DATA_BLOCK "PMA_DG1_RECV"
TITLE =
VERSION : 0.1


  STRUCT
   i_noStpULoad : BOOL ;	//Indication: No stop in case of underload
   Spare_00_1 : BOOL ;	//Spare
   Spare_00_2 : BOOL ;	//Spare
   Spare_00_3 : BOOL ;	//Spare
   Spare_00_4 : BOOL ;	//Spare
   Spare_00_5 : BOOL ;	//Spare
   Spare_00_6 : BOOL ;	//Spare
   Spare_00_7 : BOOL ;	//Spare
   i_Gen_run : BOOL ;	//Indication: DG running
   i_Gen_stp : BOOL ;	//Indication: DG not running
   i_Gen_strtAct : BOOL ;	//Indication: DG starting
   i_Gen_stpAct : BOOL ;	//Indication: DG stopping
   Spare_01_4 : BOOL ;	//Spare
   i_Gen_RdyStrt : BOOL ;	//Indication: DG ready for start
   Spare_01_6 : BOOL ;	//Spare
   Spare_01_7 : BOOL ;	//Spare
   i_GenBrkClse : BOOL ;	//Indication: Generator breaker closed
   i_GenBrkOpn : BOOL ;	//Indication: Generator breaker open
   i_GenBrkClseAct : BOOL ;	//Indication: Generator breaker closing active
   Spare_02_3 : BOOL ;	//Spare
   Spare_02_4 : BOOL ;	//Spare
   i_GenBrk_chrg : BOOL ;	//Indication: Generator spring in charge
   i_GenBrk_rdy : BOOL ;	//Indication: Generator breaker ready
   Spare_02_7 : BOOL ;	//Spare
   Spare_03_0 : BOOL ;	//Spare
   Spare_03_1 : BOOL ;	//Spare
   Spare_03_2 : BOOL ;	//Spare
   Spare_03_3 : BOOL ;	//Spare
   Spare_03_4 : BOOL ;	//Spare
   Spare_03_5 : BOOL ;	//Spare
   Spare_03_6 : BOOL ;	//Spare
   i_LifeFlag : BOOL ;	//Indication: PMS unit is alive (5sec pulse, 10 sec period)
   Spare_04_0 : BOOL ;	//Spare
   Spare_04_1 : BOOL ;	//Spare
   Spare_04_2 : BOOL ;	//Spare
   Spare_04_3 : BOOL ;	//Spare
   Spare_04_4 : BOOL ;	//Spare
   Spare_04_5 : BOOL ;	//Spare
   Spare_04_6 : BOOL ;	//Spare
   Spare_04_7 : BOOL ;	//Spare
   Spare_05_0 : BOOL ;	//Spare
   Spare_05_1 : BOOL ;	//Spare
   Spare_05_2 : BOOL ;	//Spare
   Spare_05_3 : BOOL ;	//Spare
   Spare_05_4 : BOOL ;	//Spare
   Spare_05_5 : BOOL ;	//Spare
   Spare_05_6 : BOOL ;	//Spare
   Spare_05_7 : BOOL ;	//Spare
   Spare_06_0 : BOOL ;	//Spare
   Spare_06_1 : BOOL ;	//Spare
   Spare_06_2 : BOOL ;	//Spare
   Spare_06_3 : BOOL ;	//Spare
   Spare_06_4 : BOOL ;	//Spare
   Spare_06_5 : BOOL ;	//Spare
   Spare_06_6 : BOOL ;	//Spare
   Spare_06_7 : BOOL ;	//Spare
   Spare_07_0 : BOOL ;	//Spare
   Spare_07_1 : BOOL ;	//Spare
   Spare_07_2 : BOOL ;	//Spare
   Spare_07_3 : BOOL ;	//Spare
   Spare_07_4 : BOOL ;	//Spare
   Spare_07_5 : BOOL ;	//Spare
   Spare_07_6 : BOOL ;	//Spare
   Spare_07_7 : BOOL ;	//Spare
   Spare_08_0 : BOOL ;	//Spare
   Spare_08_1 : BOOL ;	//Spare
   Spare_08_2 : BOOL ;	//Spare
   Spare_08_3 : BOOL ;	//Spare
   Spare_08_4 : BOOL ;	//Spare
   Spare_08_5 : BOOL ;	//Spare
   Spare_08_6 : BOOL ;	//Spare
   Spare_08_7 : BOOL ;	//Spare
   Spare_09_0 : BOOL ;	//Spare
   Spare_09_1 : BOOL ;	//Spare
   Spare_09_2 : BOOL ;	//Spare
   Spare_09_3 : BOOL ;	//Spare
   Spare_09_4 : BOOL ;	//Spare
   Spare_09_5 : BOOL ;	//Spare
   Spare_09_6 : BOOL ;	//Spare
   Spare_09_7 : BOOL ;	//Spare
   e_OP_err : BOOL ;	//Alarm: OP Failure
   Spare_10_1 : BOOL ;	//Spare
   e_protection_units_fail : BOOL ;	//Alarm: Protection Units Fail (Renop / Siprotec)
   Spare_10_3 : BOOL ;	//Spare
   e_MCB24_trip : BOOL ;	//Alarm: MCB DC 24V Control voltage tripped
   e_CB440G_trip : BOOL ;	//Alarm: CB AC 440V Generator voltage tripped
   e_CB440B_trip : BOOL ;	//Alarm: CB AC 440V Busbar voltage tripped
   e_InputCard : BOOL ;	//Alarm: input / output card failure
   Spare_11_0 : BOOL ;	//Spare
   Spare_11_1 : BOOL ;	//Spare
   Spare_11_2 : BOOL ;	//Spare
   e_SqChg : BOOL ;	//Alarm: Change Start/Stop Sequence not possible
   e_SetsFaded : BOOL ;	//Alarm: At least one set is out faded
   e_AutoMode : BOOL ;	//Alarm: Automatic mode is not possible
   e_StrtSqChg : BOOL ;	//Indication: Force start of 1st DG of start / stop sequence if not running
   Spare_11_7 : BOOL ;	//Spare
   e_linkT1 : BOOL ;	//Alarm: Link to tie breaker 1 faulty
   e_linkT2 : BOOL ;	//Alarm: Link to tie breaker 2 faulty
   Spare_12_2 : BOOL ;	//Spare
   Spare_12_3 : BOOL ;	//Spare
   e_linkG1 : BOOL ;	//Alarm: Link to generator 1 faulty
   e_linkG2 : BOOL ;	//Alarm: Link to generator 2 faulty
   e_linkG3 : BOOL ;	//Alarm: Link to generator 3 faulty
   e_linkG4 : BOOL ;	//Alarm: Link to generator 4 faulty
   e_linkG5 : BOOL ;	//Alarm: Link to generator 5 faulty
   e_linkG6 : BOOL ;	//Alarm: Link to generator 6 faulty
   e_linkG7 : BOOL ;	//Alarm: Link to generator 7 faulty
   e_linkG8 : BOOL ;	//Alarm: Link to generator 8 faulty
   e_linkG9 : BOOL ;	//Alarm: Link to generator 9 faulty
   Spare_13_5 : BOOL ;	//Spare
   Spare_13_6 : BOOL ;	//Spare
   Spare_13_7 : BOOL ;	//Spare
   Spare_14_0 : BOOL ;	//Spare
   Spare_14_1 : BOOL ;	//Spare
   Spare_14_2 : BOOL ;	//Spare
   Spare_14_3 : BOOL ;	//Spare
   Spare_14_4 : BOOL ;	//Spare
   Spare_14_5 : BOOL ;	//Spare
   Spare_14_6 : BOOL ;	//Spare
   Spare_14_7 : BOOL ;	//Spare
   Spare_15_0 : BOOL ;	//Spare
   Spare_15_1 : BOOL ;	//Spare
   Spare_15_2 : BOOL ;	//Spare
   Spare_15_3 : BOOL ;	//Spare
   Spare_15_4 : BOOL ;	//Spare
   Spare_15_5 : BOOL ;	//Spare
   Spare_15_6 : BOOL ;	//Spare
   Spare_15_7 : BOOL ;	//Spare
   e_Start_Fail : BOOL ;	//Alarm: DG/SG/EG start failure
   e_Stop_Fail : BOOL ;	//Alarm: DG/SG/EG stopping failure
   e_IgnSp_RelGenBrk_Fail : BOOL ;	//Alarm: Signal "Ignit. speed"/"Release gen. breaker" missing (but gen. volt. On)
   e_RatedSpeed_Fail : BOOL ;	//Alarm: Rated speed is not reached
   e_GenVolt_Fail : BOOL ;	//Alarm: Generator voltage missing (but "Ignit. speed"/"Release gen. breaker" On)
   e_DiesEngine_Fail : BOOL ;	//Alarm: Diesel engine failure
   e_Start_Fail_ext : BOOL ;	//Alarm: DG/SG/EG External start failure
   Spare_16_7 : BOOL ;	//Spare
   Spare_17_0 : BOOL ;	//Spare
   Spare_17_1 : BOOL ;	//Spare
   Spare_17_2 : BOOL ;	//Spare
   Spare_17_3 : BOOL ;	//Spare
   Spare_17_4 : BOOL ;	//Spare
   Spare_17_5 : BOOL ;	//Spare
   Spare_17_6 : BOOL ;	//Spare
   Spare_17_7 : BOOL ;	//Spare
   Spare_18_0 : BOOL ;	//Spare
   Spare_18_1 : BOOL ;	//Spare
   Spare_18_2 : BOOL ;	//Spare
   Spare_18_3 : BOOL ;	//Spare
   Spare_18_4 : BOOL ;	//Spare
   Spare_18_5 : BOOL ;	//Spare
   Spare_18_6 : BOOL ;	//Spare
   Spare_18_7 : BOOL ;	//Spare
   Spare_19_0 : BOOL ;	//Spare
   Spare_19_1 : BOOL ;	//Spare
   Spare_19_2 : BOOL ;	//Spare
   Spare_19_3 : BOOL ;	//Spare
   Spare_19_4 : BOOL ;	//Spare
   Spare_19_5 : BOOL ;	//Spare
   Spare_19_6 : BOOL ;	//Spare
   Spare_19_7 : BOOL ;	//Spare
   Spare_20_0 : BOOL ;	//Spare
   Spare_20_1 : BOOL ;	//Spare
   Spare_20_2 : BOOL ;	//Spare
   Spare_20_3 : BOOL ;	//Spare
   Spare_20_4 : BOOL ;	//Spare
   Spare_20_5 : BOOL ;	//Spare
   Spare_20_6 : BOOL ;	//Spare
   Spare_20_7 : BOOL ;	//Spare
   Spare_21_0 : BOOL ;	//Spare
   Spare_21_1 : BOOL ;	//Spare
   Spare_21_2 : BOOL ;	//Spare
   Spare_21_3 : BOOL ;	//Spare
   Spare_21_4 : BOOL ;	//Spare
   Spare_21_5 : BOOL ;	//Spare
   Spare_21_6 : BOOL ;	//Spare
   Spare_21_7 : BOOL ;	//Spare
   e_SD_C1 : BOOL ;	//Alarm: Shutdown by Engine over speed
   e_SD_C2 : BOOL ;	//Alarm: Shutdown by Engine oil presure  <<low
   e_SD_C3 : BOOL ;	//Alarm: Shutdown by Engine jaket water temperature >>high
   e_SD_C4 : BOOL ;	//Alarm: Shutdown by Engine crankcase presure >> high
   Spare_22_4 : BOOL ;	//Spare
   Spare_22_5 : BOOL ;	//Spare
   Spare_22_6 : BOOL ;	//Spare
   e_SD_C5 : BOOL ;	//Alarm: Shutdown by Engine after cooler temperature >> high
   Spare_23_0 : BOOL ;	//Spare
   Spare_23_1 : BOOL ;	//Spare
   Spare_23_2 : BOOL ;	//Spare
   Spare_23_3 : BOOL ;	//Spare
   Spare_23_4 : BOOL ;	//Spare
   Spare_23_5 : BOOL ;	//Spare
   Spare_23_6 : BOOL ;	//Spare
   Spare_23_7 : BOOL ;	//Spare
   Spare_24_0 : BOOL ;	//Spare
   Spare_24_1 : BOOL ;	//Spare
   Spare_24_2 : BOOL ;	//Spare
   Spare_24_3 : BOOL ;	//Spare
   Spare_24_4 : BOOL ;	//Spare
   Spare_24_5 : BOOL ;	//Spare
   Spare_24_6 : BOOL ;	//Spare
   Spare_24_7 : BOOL ;	//Spare
   e_EMStpMan : BOOL ;	//Alarm: Emergency stop manual
   Spare_25_1 : BOOL ;	//Spare
   Spare_25_2 : BOOL ;	//Spare
   Spare_25_3 : BOOL ;	//Spare
   Spare_25_4 : BOOL ;	//Spare
   Spare_25_5 : BOOL ;	//Spare
   Spare_25_6 : BOOL ;	//Spare
   Spare_25_7 : BOOL ;	//Spare
   e_brk_trip : BOOL ;	//Alarm: Generator breaker tripped
   e_Changeov_Blackout : BOOL ;	//Alarm: Generator breaker tripped for changeover via blackout
   e_brk_on_fail : BOOL ;	//Alarm: Generator breaker closing failure
   e_brk_off_fail : BOOL ;	//Alarm: Generator breaker opening failure
   e_brk_onOff_fail : BOOL ;	//Alarm: Plausibility failure generator breaker On / Off
   e_brk_ready_fail : BOOL ;	//Alarm: Generator breaker not ready
   e_SimLock_Fail : BOOL ;	//Alarm: Simultaneous lock time exceeded (Feedback from other gen. set missing)
   e_SynchrTime_Fail : BOOL ;	//Alarm: Synchronizing time exceeded
   Spare_27_0 : BOOL ;	//Spare
   Spare_27_1 : BOOL ;	//Spare
   e_GeneralFail : BOOL ;	//Alarm: General ciruit breaker failure
   e_DeltaVoltage : BOOL ;	//Alarm: Not permissiv voltage difference between bus bar and generator side
   e_Closed_fail : BOOL ;	//Alarm: ACB opens without command
   e_Opened_fail : BOOL ;	//Alarm: ACB closes without command
   e_Deload_fail : BOOL ;	//Alarm: Deloading faulty, ACB is opened without deloading
   Spare_27_7 : BOOL ;	//Spare
   e_Prtct_fail : BOOL ;	//Alarm: Generator protection unit failure
   e_BusBar_Monit_Fail : BOOL ;	//Alarm: Busbar monitoring failure
   e_GenVolt_Monit_Fail : BOOL ;	//Alarm: Generator voltage monitoring failure
   e_Curr_Monit_Fail : BOOL ;	//Alarm: Current monitoring failure
   Spare_28_4 : BOOL ;	//Spare
   Spare_28_5 : BOOL ;	//Spare
   Spare_28_6 : BOOL ;	//Spare
   Spare_28_7 : BOOL ;	//Spare
   e_i_SC : BOOL ;	//Alarm: Short circuit
   e_ShCirc_OtherSet : BOOL ;	//Alarm: Short circuit of other generator set (blocking of own set)
   Spare_29_2 : BOOL ;	//Spare
   e_warnCurrent2 : BOOL ;	//Warning: current limit 2 exceeded -standby start limit 2-
   e_warnCurrent3dly1 : BOOL ;	//Warning: current limit 3 exceeded -prefer.trip I- (Genop or PMS)
   e_warnCurrent3dly2 : BOOL ;	//Warning: current limit 3 exceeded -prefer.trip II- (Genop or PMS)
   e_warnCurrent3dly3 : BOOL ;	//Warning: current limit 3 exceeded -prefer.trip III- (Genop or PMS)
   e_warnCurrent61 : BOOL ;	//Warning: current limit 6 exceeded -standby start / prefer.trip I-III-
   e_GenBrkOff_Prtct : BOOL ;	//Alarm: Trip of generator breaker by overcurrent
   e_warnload1 : BOOL ;	//Warning: load limit 1 exceeded
   e_warnload2 : BOOL ;	//Warning: load limit 2 exceeded
   e_overload3 : BOOL ;	//Alarm: load limit 3 exceeded
   e_overload4 : BOOL ;	//Alarm: load limit 4 exceeded
   e_overload5 : BOOL ;	//Alarm: load limit 5 exceeded
   e_overload6 : BOOL ;	//Alarm: load limit 6 exceeded
   e_RevPower : BOOL ;	//Alarm: Trip of generator breaker by reverse power
   e_Underfrequ1 : BOOL ;	//Alarm: Standby start by underfrequency 1
   e_Underfrequ2 : BOOL ;	//Alarm: Standby start by under frequency 2
   e_Underfrequ3 : BOOL ;	//Alarm: Preferential trip I due to under frequency
   e_Underfrequ4 : BOOL ;	//Alarm: Preferential trip II due to under frequency
   e_Underfrequ5 : BOOL ;	//Alarm: Preferential trip III due to under frequency
   e_Underfrequ6 : BOOL ;	//Alarm: Common preferential trip due to under frequency
   e_Underfrequ7 : BOOL ;	//Alarm: Generator breaker trips by underfrequency
   e_Overfrequ : BOOL ;	//Alarm: Overfrequency
   e_Undervolt1 : BOOL ;	//Alarm: Change over by undervoltage 1
   e_Undervolt2 : BOOL ;	//Alarm: Trip of generator breaker by undervoltage 2
   e_Overvolt1 : BOOL ;	//Alarm: Change over by Overvoltage 1
   e_Overvolt2 : BOOL ;	//Alarm: Trip of generator breaker by overvoltage 2 (plus deexitation)
   e_Overvolt3 : BOOL ;	//Alarm: Trip of generator breaker by overvoltage 3 (plus deexitation)
   Spare_32_5 : BOOL ;	//Spare
   e_warnReactPwr1 : BOOL ;	//Warning: re-active power limit 1 exceeded
   Spare_32_7 : BOOL ;	//Spare
   Spare_33_0 : BOOL ;	//Spare
   Spare_33_1 : BOOL ;	//Spare
   e_DiffProt_Trip : BOOL ;	//Alarm: Trip of generator breaker by differential protection
   Spare_33_3 : BOOL ;	//Spare
   Spare_33_4 : BOOL ;	//Spare
   Spare_33_5 : BOOL ;	//Spare
   e_ComTripExtDevice : BOOL ;	//Alarm: Common trip external device
   Spare_33_7 : BOOL ;	//Spare
   Spare_34_0 : BOOL ;	//Spare
   Spare_34_1 : BOOL ;	//Spare
   Spare_34_2 : BOOL ;	//Spare
   Spare_34_3 : BOOL ;	//Spare
   Spare_34_4 : BOOL ;	//Spare
   Spare_34_5 : BOOL ;	//Spare
   Spare_34_6 : BOOL ;	//Spare
   Spare_34_7 : BOOL ;	//Spare
   Spare_35_0 : BOOL ;	//Spare
   Spare_35_1 : BOOL ;	//Spare
   Spare_35_2 : BOOL ;	//Spare
   Spare_35_3 : BOOL ;	//Spare
   Spare_35_4 : BOOL ;	//Spare
   Spare_35_5 : BOOL ;	//Spare
   Spare_35_6 : BOOL ;	//Spare
   Spare_35_7 : BOOL ;	//Spare
   e_CB_ContrVolt : BOOL ;	//Alarm: CB control voltage fault
   Spare_36_1 : BOOL ;	//Spare
   Spare_36_2 : BOOL ;	//Spare
   Spare_36_3 : BOOL ;	//Spare
   e_CB_Earthed : BOOL ;	//Alarm: CB earthed
   Spare_36_5 : BOOL ;	//Spare
   Spare_36_6 : BOOL ;	//Spare
   Spare_36_7 : BOOL ;	//Spare
   i_AutoStopPreInd : BOOL ;	//Indication: Underload shutdown, annunciation
   i_AutoStop : BOOL ;	//Indication: Underload shutdown, activation
   e_StopNotPermit : BOOL ;	//Alarm: Stop via pushbutton in automatic not permitted
   i_LoadTooLow : BOOL ;	//Indication: Load too low for generator set (if SG the last Set on busbar)
   e_StStart : BOOL ;	//Indication: Standby start by overcurrent, overload, etc.
   e_StStartNoPos : BOOL ;	//Alarm: Standby start not possible
   e_2ndStStart : BOOL ;	//Indication: 2nd Standby start by overcurrent, overload, etc.
   e_2ndStStartNoPos : BOOL ;	//Alarm: 2nd Standby start not possible
   Spare_38_0 : BOOL ;	//Spare
   Spare_38_1 : BOOL ;	//Spare
   Spare_38_2 : BOOL ;	//Spare
   Spare_38_3 : BOOL ;	//Spare
   Spare_38_4 : BOOL ;	//Spare
   Spare_38_5 : BOOL ;	//Spare
   Spare_38_6 : BOOL ;	//Spare
   Spare_38_7 : BOOL ;	//Spare
   e_NoSetsAvailMM : BOOL ;	//Alarm "No set available"
   e_StandbyStartMM : BOOL ;	//Alarm "Failure standby start" Minimum sets
   e_NoSetsAutoMM : BOOL ;	//Alarm "No set in automatic, stop not possible" Maximum sets
   e_StoppingMM : BOOL ;	//Alarm "Failure stopping of set" Maximum sets
   e_StStartMinSets : BOOL ;	//Ind: Standby start due to selected minimum sets
   e_ACBoffNotPermit : BOOL ;	//Alarm: ACB off via pushbutton is not permitted
   e_Limitation : BOOL ;	//Alarm: Selected limitation has been exceeded
   Spare_39_7 : BOOL ;	//Spare
   e_deviL_FCtrl : BOOL ;	//Alarm: Not aceptable deviation Load-/Frequency controller
   Spare_40_1 : BOOL ;	//Spare
   Spare_40_2 : BOOL ;	//Spare
   Spare_40_3 : BOOL ;	//Spare
   Spare_40_4 : BOOL ;	//Spare
   Spare_40_5 : BOOL ;	//Spare
   Spare_40_6 : BOOL ;	//Spare
   Spare_40_7 : BOOL ;	//Spare
   Spare_41_0 : BOOL ;	//Spare
   Spare_41_1 : BOOL ;	//Spare
   Spare_41_2 : BOOL ;	//Spare
   Spare_41_3 : BOOL ;	//Spare
   Spare_41_4 : BOOL ;	//Spare
   Spare_41_5 : BOOL ;	//Spare
   Spare_41_6 : BOOL ;	//Spare
   Spare_41_7 : BOOL ;	//Spare
   Spare_42_0 : BOOL ;	//Spare
   Spare_42_1 : BOOL ;	//Spare
   Spare_42_2 : BOOL ;	//Spare
   Spare_42_3 : BOOL ;	//Spare
   Spare_42_4 : BOOL ;	//Spare
   Spare_42_5 : BOOL ;	//Spare
   Spare_42_6 : BOOL ;	//Spare
   Spare_42_7 : BOOL ;	//Spare
   Spare_43_0 : BOOL ;	//Spare
   Spare_43_1 : BOOL ;	//Spare
   Spare_43_2 : BOOL ;	//Spare
   Spare_43_3 : BOOL ;	//Spare
   Spare_43_4 : BOOL ;	//Spare
   Spare_43_5 : BOOL ;	//Spare
   Spare_43_6 : BOOL ;	//Spare
   Spare_43_7 : BOOL ;	//Spare
   Spare_44_0 : BOOL ;	//Spare
   Spare_44_1 : BOOL ;	//Spare
   Spare_44_2 : BOOL ;	//Spare
   Spare_44_3 : BOOL ;	//Spare
   Spare_44_4 : BOOL ;	//Spare
   Spare_44_5 : BOOL ;	//Spare
   Spare_44_6 : BOOL ;	//Spare
   Spare_44_7 : BOOL ;	//Spare
   Spare_45_0 : BOOL ;	//Spare
   Spare_45_1 : BOOL ;	//Spare
   Spare_45_2 : BOOL ;	//Spare
   Spare_45_3 : BOOL ;	//Spare
   Spare_45_4 : BOOL ;	//Spare
   Spare_45_5 : BOOL ;	//Spare
   Spare_45_6 : BOOL ;	//Spare
   Spare_45_7 : BOOL ;	//Spare
   Spare_46_0 : BOOL ;	//Spare
   Spare_46_1 : BOOL ;	//Spare
   Spare_46_2 : BOOL ;	//Spare
   Spare_46_3 : BOOL ;	//Spare
   Spare_46_4 : BOOL ;	//Spare
   Spare_46_5 : BOOL ;	//Spare
   Spare_46_6 : BOOL ;	//Spare
   Spare_46_7 : BOOL ;	//Spare
   Spare_47_0 : BOOL ;	//Spare
   Spare_47_1 : BOOL ;	//Spare
   Spare_47_2 : BOOL ;	//Spare
   Spare_47_3 : BOOL ;	//Spare
   Spare_47_4 : BOOL ;	//Spare
   Spare_47_5 : BOOL ;	//Spare
   Spare_47_6 : BOOL ;	//Spare
   Spare_47_7 : BOOL ;	//Spare
   Spare_48_0 : BOOL ;	//Spare
   Spare_48_1 : BOOL ;	//Spare
   Spare_48_2 : BOOL ;	//Spare
   Spare_48_3 : BOOL ;	//Spare
   Spare_48_4 : BOOL ;	//Spare
   Spare_48_5 : BOOL ;	//Spare
   Spare_48_6 : BOOL ;	//Spare
   Spare_48_7 : BOOL ;	//Spare
   Spare_49_0 : BOOL ;	//Spare
   Spare_49_1 : BOOL ;	//Spare
   Spare_49_2 : BOOL ;	//Spare
   Spare_49_3 : BOOL ;	//Spare
   Spare_49_4 : BOOL ;	//Spare
   Spare_49_5 : BOOL ;	//Spare
   Spare_49_6 : BOOL ;	//Spare
   Spare_49_7 : BOOL ;	//Spare
   Spare_50_0 : BOOL ;	//Spare
   Spare_50_1 : BOOL ;	//Spare
   Spare_50_2 : BOOL ;	//Spare
   Spare_50_3 : BOOL ;	//Spare
   Spare_50_4 : BOOL ;	//Spare
   Spare_50_5 : BOOL ;	//Spare
   Spare_50_6 : BOOL ;	//Spare
   Spare_50_7 : BOOL ;	//Spare
   Spare_51_0 : BOOL ;	//Spare
   Spare_51_1 : BOOL ;	//Spare
   Spare_51_2 : BOOL ;	//Spare
   Spare_51_3 : BOOL ;	//Spare
   Spare_51_4 : BOOL ;	//Spare
   Spare_51_5 : BOOL ;	//Spare
   Spare_51_6 : BOOL ;	//Spare
   Spare_51_7 : BOOL ;	//Spare
   Spare_52_0 : BOOL ;	//Spare
   Spare_52_1 : BOOL ;	//Spare
   Spare_52_2 : BOOL ;	//Spare
   Spare_52_3 : BOOL ;	//Spare
   Spare_52_4 : BOOL ;	//Spare
   Spare_52_5 : BOOL ;	//Spare
   Spare_52_6 : BOOL ;	//Spare
   Spare_52_7 : BOOL ;	//Spare
   Spare_53_0 : BOOL ;	//Spare
   Spare_53_1 : BOOL ;	//Spare
   Spare_53_2 : BOOL ;	//Spare
   Spare_53_3 : BOOL ;	//Spare
   Spare_53_4 : BOOL ;	//Spare
   Spare_53_5 : BOOL ;	//Spare
   Spare_53_6 : BOOL ;	//Spare
   Spare_53_7 : BOOL ;	//Spare
   Spare_54_0 : BOOL ;	//Spare
   Spare_54_1 : BOOL ;	//Spare
   Spare_54_2 : BOOL ;	//Spare
   Spare_54_3 : BOOL ;	//Spare
   Spare_54_4 : BOOL ;	//Spare
   Spare_54_5 : BOOL ;	//Spare
   Spare_54_6 : BOOL ;	//Spare
   Spare_54_7 : BOOL ;	//Spare
   Spare_55_0 : BOOL ;	//Spare
   Spare_55_1 : BOOL ;	//Spare
   Spare_55_2 : BOOL ;	//Spare
   Spare_55_3 : BOOL ;	//Spare
   Spare_55_4 : BOOL ;	//Spare
   Spare_55_5 : BOOL ;	//Spare
   Spare_55_6 : BOOL ;	//Spare
   Spare_55_7 : BOOL ;	//Spare
   Spare_56_0 : BOOL ;	//Spare
   Spare_56_1 : BOOL ;	//Spare
   Spare_56_2 : BOOL ;	//Spare
   Spare_56_3 : BOOL ;	//Spare
   Spare_56_4 : BOOL ;	//Spare
   Spare_56_5 : BOOL ;	//Spare
   Spare_56_6 : BOOL ;	//Spare
   Spare_56_7 : BOOL ;	//Spare
   Spare_57_0 : BOOL ;	//Spare
   Spare_57_1 : BOOL ;	//Spare
   Spare_57_2 : BOOL ;	//Spare
   Spare_57_3 : BOOL ;	//Spare
   Spare_57_4 : BOOL ;	//Spare
   Spare_57_5 : BOOL ;	//Spare
   Spare_57_6 : BOOL ;	//Spare
   Spare_57_7 : BOOL ;	//Spare
   Spare_58_0 : BOOL ;	//Spare
   Spare_58_1 : BOOL ;	//Spare
   Spare_58_2 : BOOL ;	//Spare
   Spare_58_3 : BOOL ;	//Spare
   Spare_58_4 : BOOL ;	//Spare
   Spare_58_5 : BOOL ;	//Spare
   Spare_58_6 : BOOL ;	//Spare
   Spare_58_7 : BOOL ;	//Spare
   Spare_59_0 : BOOL ;	//Spare
   Spare_59_1 : BOOL ;	//Spare
   Spare_59_2 : BOOL ;	//Spare
   Spare_59_3 : BOOL ;	//Spare
   Spare_59_4 : BOOL ;	//Spare
   Spare_59_5 : BOOL ;	//Spare
   Spare_59_6 : BOOL ;	//Spare
   Spare_59_7 : BOOL ;	//Spare
   Spare_60 : INT ;	//Spare
   Spare_62 : INT ;	//Spare
   Spare_64 : INT ;	//Spare
   Spare_66 : INT ;	//Spare
   Spare_68 : INT ;	//Spare
   Spare_70 : INT ;	//Spare
   Spare_72 : INT ;	//Spare
   Spare_74 : INT ;	//Spare
   Spare_76 : INT ;	//Spare
   Spare_78 : INT ;	//Spare
   Spare_80 : INT ;	//Spare
   Spare_82 : INT ;	//Spare
   Spare_84 : INT ;	//Spare
   Spare_86 : INT ;	//Spare
   Spare_88 : INT ;	//Spare
   Spare_90 : INT ;	//Spare
   Spare_92 : INT ;	//Spare
   Spare_94 : INT ;	//Spare
   Spare_96 : INT ;	//Spare
   Spare_98 : INT ;	//Spare
   Spare_100 : INT ;	//Spare
   Spare_102 : INT ;	//Spare
   Spare_104 : INT ;	//Spare
   Spare_106 : INT ;	//Spare
   Spare_108 : INT ;	//Spare
   Spare_110 : INT ;	//Spare
   Spare_112 : INT ;	//Spare
   Spare_114 : INT ;	//Spare
   Spare_116 : INT ;	//Spare
   Spare_118 : INT ;	//Spare
   Spare_120 : INT ;	//Spare
   Spare_122 : INT ;	//Spare
   Spare_124 : INT ;	//Spare
   Spare_126 : INT ;	//Spare
   Spare_128 : INT ;	//Spare
   Spare_130 : INT ;	//Spare
   Spare_132 : INT ;	//Spare
   Spare_134 : INT ;	//Spare
   Spare_136 : INT ;	//Spare
   Spare_138 : INT ;	//Spare
   Spare_140 : INT ;	//Spare
   Spare_142 : INT ;	//Spare
   Spare_144 : INT ;	//Spare
   Spare_146 : INT ;	//Spare
   Spare_148 : INT ;	//Spare
   Spare_150 : INT ;	//Spare
   Spare_152 : INT ;	//Spare
   Spare_154 : INT ;	//Spare
   Spare_156 : INT ;	//Spare
   Spare_158 : INT ;	//Spare
   Spare_160 : INT ;	//Spare
   Spare_162 : INT ;	//Spare
   Spare_164 : INT ;	//Spare
   Spare_166 : INT ;	//Spare
   Spare_168 : INT ;	//Spare
   Spare_170 : INT ;	//Spare
   Spare_172 : INT ;	//Spare
   Spare_174 : INT ;	//Spare
   Spare_176 : INT ;	//Spare
   Spare_178 : INT ;	//Spare
   Spare_180 : INT ;	//Spare
   Spare_182 : INT ;	//Spare
   Spare_184 : INT ;	//Spare
   Spare_186 : INT ;	//Spare
   Spare_188 : INT ;	//Spare
   Spare_190 : INT ;	//Spare
   Spare_192 : INT ;	//Spare
   Spare_194 : INT ;	//Spare
   Spare_196 : INT ;	//Spare
   Spare_198 : INT ;	//Spare
   Spare_200 : INT ;	//Spare
   Spare_202 : INT ;	//Spare
   Spare_204 : INT ;	//Spare
   Spare_206 : INT ;	//Spare
   Spare_208 : INT ;	//Spare
   Spare_210 : INT ;	//Spare
   Spare_212 : INT ;	//Spare
   Spare_214 : INT ;	//Spare
   Spare_216 : INT ;	//Spare
   Spare_218 : INT ;	//Spare
   Spare_220 : INT ;	//Spare
   Spare_222 : INT ;	//Spare
   Spare_224 : INT ;	//Spare
   Spare_226 : INT ;	//Spare
   Spare_228 : INT ;	//Spare
   Spare_230 : INT ;	//Spare
   Spare_232 : INT ;	//Spare
   Spare_234 : INT ;	//Spare
   Spare_236 : INT ;	//Spare
   Spare_238 : INT ;	//Spare
   Spare_240 : INT ;	//Spare
   Spare_242 : INT ;	//Spare
   Spare_244 : INT ;	//Spare
   Spare_246 : INT ;	//Spare
   Spare_248 : INT ;	//Spare
   Spare_250 : INT ;	//Spare
   Spare_252 : INT ;	//Spare
   Spare_254 : INT ;	//Spare
   Spare_256 : INT ;	//Spare
   Spare_258 : INT ;	//Spare
   Spare_260 : INT ;	//Spare
   Spare_262 : INT ;	//Spare
   Spare_264 : INT ;	//Spare
   Spare_266 : INT ;	//Spare
   Spare_268 : INT ;	//Spare
   Spare_270 : INT ;	//Spare
   Spare_272 : INT ;	//Spare
   Spare_274 : INT ;	//Spare
   Spare_276 : INT ;	//Spare
   Spare_278 : INT ;	//Spare
   Spare_280 : INT ;	//Spare
   Spare_282 : INT ;	//Spare
   Spare_284 : INT ;	//Spare
   Spare_286 : INT ;	//Spare
   Spare_288 : INT ;	//Spare
   Spare_290 : INT ;	//Spare
   Spare_292 : INT ;	//Spare
   Spare_294 : INT ;	//Spare
   Spare_296 : INT ;	//Spare
   Spare_298 : INT ;	//Spare
  END_STRUCT ;
BEGIN
   i_noStpULoad := FALSE;
   Spare_00_1 := FALSE;
   Spare_00_2 := FALSE;
   Spare_00_3 := FALSE;
   Spare_00_4 := FALSE;
   Spare_00_5 := FALSE;
   Spare_00_6 := FALSE;
   Spare_00_7 := FALSE;
   i_Gen_run := FALSE;
   i_Gen_stp := FALSE;
   i_Gen_strtAct := FALSE;
   i_Gen_stpAct := FALSE;
   Spare_01_4 := FALSE;
   i_Gen_RdyStrt := FALSE;
   Spare_01_6 := FALSE;
   Spare_01_7 := FALSE;
   i_GenBrkClse := FALSE;
   i_GenBrkOpn := FALSE;
   i_GenBrkClseAct := FALSE;
   Spare_02_3 := FALSE;
   Spare_02_4 := FALSE;
   i_GenBrk_chrg := FALSE;
   i_GenBrk_rdy := FALSE;
   Spare_02_7 := FALSE;
   Spare_03_0 := FALSE;
   Spare_03_1 := FALSE;
   Spare_03_2 := FALSE;
   Spare_03_3 := FALSE;
   Spare_03_4 := FALSE;
   Spare_03_5 := FALSE;
   Spare_03_6 := FALSE;
   i_LifeFlag := FALSE;
   Spare_04_0 := FALSE;
   Spare_04_1 := FALSE;
   Spare_04_2 := FALSE;
   Spare_04_3 := FALSE;
   Spare_04_4 := FALSE;
   Spare_04_5 := FALSE;
   Spare_04_6 := FALSE;
   Spare_04_7 := FALSE;
   Spare_05_0 := FALSE;
   Spare_05_1 := FALSE;
   Spare_05_2 := FALSE;
   Spare_05_3 := FALSE;
   Spare_05_4 := FALSE;
   Spare_05_5 := FALSE;
   Spare_05_6 := FALSE;
   Spare_05_7 := FALSE;
   Spare_06_0 := FALSE;
   Spare_06_1 := FALSE;
   Spare_06_2 := FALSE;
   Spare_06_3 := FALSE;
   Spare_06_4 := FALSE;
   Spare_06_5 := FALSE;
   Spare_06_6 := FALSE;
   Spare_06_7 := FALSE;
   Spare_07_0 := FALSE;
   Spare_07_1 := FALSE;
   Spare_07_2 := FALSE;
   Spare_07_3 := FALSE;
   Spare_07_4 := FALSE;
   Spare_07_5 := FALSE;
   Spare_07_6 := FALSE;
   Spare_07_7 := FALSE;
   Spare_08_0 := FALSE;
   Spare_08_1 := FALSE;
   Spare_08_2 := FALSE;
   Spare_08_3 := FALSE;
   Spare_08_4 := FALSE;
   Spare_08_5 := FALSE;
   Spare_08_6 := FALSE;
   Spare_08_7 := FALSE;
   Spare_09_0 := FALSE;
   Spare_09_1 := FALSE;
   Spare_09_2 := FALSE;
   Spare_09_3 := FALSE;
   Spare_09_4 := FALSE;
   Spare_09_5 := FALSE;
   Spare_09_6 := FALSE;
   Spare_09_7 := FALSE;
   e_OP_err := FALSE;
   Spare_10_1 := FALSE;
   e_protection_units_fail := FALSE;
   Spare_10_3 := FALSE;
   e_MCB24_trip := FALSE;
   e_CB440G_trip := FALSE;
   e_CB440B_trip := FALSE;
   e_InputCard := FALSE;
   Spare_11_0 := FALSE;
   Spare_11_1 := FALSE;
   Spare_11_2 := FALSE;
   e_SqChg := FALSE;
   e_SetsFaded := FALSE;
   e_AutoMode := FALSE;
   e_StrtSqChg := FALSE;
   Spare_11_7 := FALSE;
   e_linkT1 := FALSE;
   e_linkT2 := FALSE;
   Spare_12_2 := FALSE;
   Spare_12_3 := FALSE;
   e_linkG1 := FALSE;
   e_linkG2 := FALSE;
   e_linkG3 := FALSE;
   e_linkG4 := FALSE;
   e_linkG5 := FALSE;
   e_linkG6 := FALSE;
   e_linkG7 := FALSE;
   e_linkG8 := FALSE;
   e_linkG9 := FALSE;
   Spare_13_5 := FALSE;
   Spare_13_6 := FALSE;
   Spare_13_7 := FALSE;
   Spare_14_0 := FALSE;
   Spare_14_1 := FALSE;
   Spare_14_2 := FALSE;
   Spare_14_3 := FALSE;
   Spare_14_4 := FALSE;
   Spare_14_5 := FALSE;
   Spare_14_6 := FALSE;
   Spare_14_7 := FALSE;
   Spare_15_0 := FALSE;
   Spare_15_1 := FALSE;
   Spare_15_2 := FALSE;
   Spare_15_3 := FALSE;
   Spare_15_4 := FALSE;
   Spare_15_5 := FALSE;
   Spare_15_6 := FALSE;
   Spare_15_7 := FALSE;
   e_Start_Fail := FALSE;
   e_Stop_Fail := FALSE;
   e_IgnSp_RelGenBrk_Fail := FALSE;
   e_RatedSpeed_Fail := FALSE;
   e_GenVolt_Fail := FALSE;
   e_DiesEngine_Fail := FALSE;
   e_Start_Fail_ext := FALSE;
   Spare_16_7 := FALSE;
   Spare_17_0 := FALSE;
   Spare_17_1 := FALSE;
   Spare_17_2 := FALSE;
   Spare_17_3 := FALSE;
   Spare_17_4 := FALSE;
   Spare_17_5 := FALSE;
   Spare_17_6 := FALSE;
   Spare_17_7 := FALSE;
   Spare_18_0 := FALSE;
   Spare_18_1 := FALSE;
   Spare_18_2 := FALSE;
   Spare_18_3 := FALSE;
   Spare_18_4 := FALSE;
   Spare_18_5 := FALSE;
   Spare_18_6 := FALSE;
   Spare_18_7 := FALSE;
   Spare_19_0 := FALSE;
   Spare_19_1 := FALSE;
   Spare_19_2 := FALSE;
   Spare_19_3 := FALSE;
   Spare_19_4 := FALSE;
   Spare_19_5 := FALSE;
   Spare_19_6 := FALSE;
   Spare_19_7 := FALSE;
   Spare_20_0 := FALSE;
   Spare_20_1 := FALSE;
   Spare_20_2 := FALSE;
   Spare_20_3 := FALSE;
   Spare_20_4 := FALSE;
   Spare_20_5 := FALSE;
   Spare_20_6 := FALSE;
   Spare_20_7 := FALSE;
   Spare_21_0 := FALSE;
   Spare_21_1 := FALSE;
   Spare_21_2 := FALSE;
   Spare_21_3 := FALSE;
   Spare_21_4 := FALSE;
   Spare_21_5 := FALSE;
   Spare_21_6 := FALSE;
   Spare_21_7 := FALSE;
   e_SD_C1 := FALSE;
   e_SD_C2 := FALSE;
   e_SD_C3 := FALSE;
   e_SD_C4 := FALSE;
   Spare_22_4 := FALSE;
   Spare_22_5 := FALSE;
   Spare_22_6 := FALSE;
   e_SD_C5 := FALSE;
   Spare_23_0 := FALSE;
   Spare_23_1 := FALSE;
   Spare_23_2 := FALSE;
   Spare_23_3 := FALSE;
   Spare_23_4 := FALSE;
   Spare_23_5 := FALSE;
   Spare_23_6 := FALSE;
   Spare_23_7 := FALSE;
   Spare_24_0 := FALSE;
   Spare_24_1 := FALSE;
   Spare_24_2 := FALSE;
   Spare_24_3 := FALSE;
   Spare_24_4 := FALSE;
   Spare_24_5 := FALSE;
   Spare_24_6 := FALSE;
   Spare_24_7 := FALSE;
   e_EMStpMan := FALSE;
   Spare_25_1 := FALSE;
   Spare_25_2 := FALSE;
   Spare_25_3 := FALSE;
   Spare_25_4 := FALSE;
   Spare_25_5 := FALSE;
   Spare_25_6 := FALSE;
   Spare_25_7 := FALSE;
   e_brk_trip := FALSE;
   e_Changeov_Blackout := FALSE;
   e_brk_on_fail := FALSE;
   e_brk_off_fail := FALSE;
   e_brk_onOff_fail := FALSE;
   e_brk_ready_fail := FALSE;
   e_SimLock_Fail := FALSE;
   e_SynchrTime_Fail := FALSE;
   Spare_27_0 := FALSE;
   Spare_27_1 := FALSE;
   e_GeneralFail := FALSE;
   e_DeltaVoltage := FALSE;
   e_Closed_fail := FALSE;
   e_Opened_fail := FALSE;
   e_Deload_fail := FALSE;
   Spare_27_7 := FALSE;
   e_Prtct_fail := FALSE;
   e_BusBar_Monit_Fail := FALSE;
   e_GenVolt_Monit_Fail := FALSE;
   e_Curr_Monit_Fail := FALSE;
   Spare_28_4 := FALSE;
   Spare_28_5 := FALSE;
   Spare_28_6 := FALSE;
   Spare_28_7 := FALSE;
   e_i_SC := FALSE;
   e_ShCirc_OtherSet := FALSE;
   Spare_29_2 := FALSE;
   e_warnCurrent2 := FALSE;
   e_warnCurrent3dly1 := FALSE;
   e_warnCurrent3dly2 := FALSE;
   e_warnCurrent3dly3 := FALSE;
   e_warnCurrent61 := FALSE;
   e_GenBrkOff_Prtct := FALSE;
   e_warnload1 := FALSE;
   e_warnload2 := FALSE;
   e_overload3 := FALSE;
   e_overload4 := FALSE;
   e_overload5 := FALSE;
   e_overload6 := FALSE;
   e_RevPower := FALSE;
   e_Underfrequ1 := FALSE;
   e_Underfrequ2 := FALSE;
   e_Underfrequ3 := FALSE;
   e_Underfrequ4 := FALSE;
   e_Underfrequ5 := FALSE;
   e_Underfrequ6 := FALSE;
   e_Underfrequ7 := FALSE;
   e_Overfrequ := FALSE;
   e_Undervolt1 := FALSE;
   e_Undervolt2 := FALSE;
   e_Overvolt1 := FALSE;
   e_Overvolt2 := FALSE;
   e_Overvolt3 := FALSE;
   Spare_32_5 := FALSE;
   e_warnReactPwr1 := FALSE;
   Spare_32_7 := FALSE;
   Spare_33_0 := FALSE;
   Spare_33_1 := FALSE;
   e_DiffProt_Trip := FALSE;
   Spare_33_3 := FALSE;
   Spare_33_4 := FALSE;
   Spare_33_5 := FALSE;
   e_ComTripExtDevice := FALSE;
   Spare_33_7 := FALSE;
   Spare_34_0 := FALSE;
   Spare_34_1 := FALSE;
   Spare_34_2 := FALSE;
   Spare_34_3 := FALSE;
   Spare_34_4 := FALSE;
   Spare_34_5 := FALSE;
   Spare_34_6 := FALSE;
   Spare_34_7 := FALSE;
   Spare_35_0 := FALSE;
   Spare_35_1 := FALSE;
   Spare_35_2 := FALSE;
   Spare_35_3 := FALSE;
   Spare_35_4 := FALSE;
   Spare_35_5 := FALSE;
   Spare_35_6 := FALSE;
   Spare_35_7 := FALSE;
   e_CB_ContrVolt := FALSE;
   Spare_36_1 := FALSE;
   Spare_36_2 := FALSE;
   Spare_36_3 := FALSE;
   e_CB_Earthed := FALSE;
   Spare_36_5 := FALSE;
   Spare_36_6 := FALSE;
   Spare_36_7 := FALSE;
   i_AutoStopPreInd := FALSE;
   i_AutoStop := FALSE;
   e_StopNotPermit := FALSE;
   i_LoadTooLow := FALSE;
   e_StStart := FALSE;
   e_StStartNoPos := FALSE;
   e_2ndStStart := FALSE;
   e_2ndStStartNoPos := FALSE;
   Spare_38_0 := FALSE;
   Spare_38_1 := FALSE;
   Spare_38_2 := FALSE;
   Spare_38_3 := FALSE;
   Spare_38_4 := FALSE;
   Spare_38_5 := FALSE;
   Spare_38_6 := FALSE;
   Spare_38_7 := FALSE;
   e_NoSetsAvailMM := FALSE;
   e_StandbyStartMM := FALSE;
   e_NoSetsAutoMM := FALSE;
   e_StoppingMM := FALSE;
   e_StStartMinSets := FALSE;
   e_ACBoffNotPermit := FALSE;
   e_Limitation := FALSE;
   Spare_39_7 := FALSE;
   e_deviL_FCtrl := FALSE;
   Spare_40_1 := FALSE;
   Spare_40_2 := FALSE;
   Spare_40_3 := FALSE;
   Spare_40_4 := FALSE;
   Spare_40_5 := FALSE;
   Spare_40_6 := FALSE;
   Spare_40_7 := FALSE;
   Spare_41_0 := FALSE;
   Spare_41_1 := FALSE;
   Spare_41_2 := FALSE;
   Spare_41_3 := FALSE;
   Spare_41_4 := FALSE;
   Spare_41_5 := FALSE;
   Spare_41_6 := FALSE;
   Spare_41_7 := FALSE;
   Spare_42_0 := FALSE;
   Spare_42_1 := FALSE;
   Spare_42_2 := FALSE;
   Spare_42_3 := FALSE;
   Spare_42_4 := FALSE;
   Spare_42_5 := FALSE;
   Spare_42_6 := FALSE;
   Spare_42_7 := FALSE;
   Spare_43_0 := FALSE;
   Spare_43_1 := FALSE;
   Spare_43_2 := FALSE;
   Spare_43_3 := FALSE;
   Spare_43_4 := FALSE;
   Spare_43_5 := FALSE;
   Spare_43_6 := FALSE;
   Spare_43_7 := FALSE;
   Spare_44_0 := FALSE;
   Spare_44_1 := FALSE;
   Spare_44_2 := FALSE;
   Spare_44_3 := FALSE;
   Spare_44_4 := FALSE;
   Spare_44_5 := FALSE;
   Spare_44_6 := FALSE;
   Spare_44_7 := FALSE;
   Spare_45_0 := FALSE;
   Spare_45_1 := FALSE;
   Spare_45_2 := FALSE;
   Spare_45_3 := FALSE;
   Spare_45_4 := FALSE;
   Spare_45_5 := FALSE;
   Spare_45_6 := FALSE;
   Spare_45_7 := FALSE;
   Spare_46_0 := FALSE;
   Spare_46_1 := FALSE;
   Spare_46_2 := FALSE;
   Spare_46_3 := FALSE;
   Spare_46_4 := FALSE;
   Spare_46_5 := FALSE;
   Spare_46_6 := FALSE;
   Spare_46_7 := FALSE;
   Spare_47_0 := FALSE;
   Spare_47_1 := FALSE;
   Spare_47_2 := FALSE;
   Spare_47_3 := FALSE;
   Spare_47_4 := FALSE;
   Spare_47_5 := FALSE;
   Spare_47_6 := FALSE;
   Spare_47_7 := FALSE;
   Spare_48_0 := FALSE;
   Spare_48_1 := FALSE;
   Spare_48_2 := FALSE;
   Spare_48_3 := FALSE;
   Spare_48_4 := FALSE;
   Spare_48_5 := FALSE;
   Spare_48_6 := FALSE;
   Spare_48_7 := FALSE;
   Spare_49_0 := FALSE;
   Spare_49_1 := FALSE;
   Spare_49_2 := FALSE;
   Spare_49_3 := FALSE;
   Spare_49_4 := FALSE;
   Spare_49_5 := FALSE;
   Spare_49_6 := FALSE;
   Spare_49_7 := FALSE;
   Spare_50_0 := FALSE;
   Spare_50_1 := FALSE;
   Spare_50_2 := FALSE;
   Spare_50_3 := FALSE;
   Spare_50_4 := FALSE;
   Spare_50_5 := FALSE;
   Spare_50_6 := FALSE;
   Spare_50_7 := FALSE;
   Spare_51_0 := FALSE;
   Spare_51_1 := FALSE;
   Spare_51_2 := FALSE;
   Spare_51_3 := FALSE;
   Spare_51_4 := FALSE;
   Spare_51_5 := FALSE;
   Spare_51_6 := FALSE;
   Spare_51_7 := FALSE;
   Spare_52_0 := FALSE;
   Spare_52_1 := FALSE;
   Spare_52_2 := FALSE;
   Spare_52_3 := FALSE;
   Spare_52_4 := FALSE;
   Spare_52_5 := FALSE;
   Spare_52_6 := FALSE;
   Spare_52_7 := FALSE;
   Spare_53_0 := FALSE;
   Spare_53_1 := FALSE;
   Spare_53_2 := FALSE;
   Spare_53_3 := FALSE;
   Spare_53_4 := FALSE;
   Spare_53_5 := FALSE;
   Spare_53_6 := FALSE;
   Spare_53_7 := FALSE;
   Spare_54_0 := FALSE;
   Spare_54_1 := FALSE;
   Spare_54_2 := FALSE;
   Spare_54_3 := FALSE;
   Spare_54_4 := FALSE;
   Spare_54_5 := FALSE;
   Spare_54_6 := FALSE;
   Spare_54_7 := FALSE;
   Spare_55_0 := FALSE;
   Spare_55_1 := FALSE;
   Spare_55_2 := FALSE;
   Spare_55_3 := FALSE;
   Spare_55_4 := FALSE;
   Spare_55_5 := FALSE;
   Spare_55_6 := FALSE;
   Spare_55_7 := FALSE;
   Spare_56_0 := FALSE;
   Spare_56_1 := FALSE;
   Spare_56_2 := FALSE;
   Spare_56_3 := FALSE;
   Spare_56_4 := FALSE;
   Spare_56_5 := FALSE;
   Spare_56_6 := FALSE;
   Spare_56_7 := FALSE;
   Spare_57_0 := FALSE;
   Spare_57_1 := FALSE;
   Spare_57_2 := FALSE;
   Spare_57_3 := FALSE;
   Spare_57_4 := FALSE;
   Spare_57_5 := FALSE;
   Spare_57_6 := FALSE;
   Spare_57_7 := FALSE;
   Spare_58_0 := FALSE;
   Spare_58_1 := FALSE;
   Spare_58_2 := FALSE;
   Spare_58_3 := FALSE;
   Spare_58_4 := FALSE;
   Spare_58_5 := FALSE;
   Spare_58_6 := FALSE;
   Spare_58_7 := FALSE;
   Spare_59_0 := FALSE;
   Spare_59_1 := FALSE;
   Spare_59_2 := FALSE;
   Spare_59_3 := FALSE;
   Spare_59_4 := FALSE;
   Spare_59_5 := FALSE;
   Spare_59_6 := FALSE;
   Spare_59_7 := FALSE;
   Spare_60 := 0;
   Spare_62 := 0;
   Spare_64 := 0;
   Spare_66 := 0;
   Spare_68 := 0;
   Spare_70 := 0;
   Spare_72 := 0;
   Spare_74 := 0;
   Spare_76 := 0;
   Spare_78 := 0;
   Spare_80 := 0;
   Spare_82 := 0;
   Spare_84 := 0;
   Spare_86 := 0;
   Spare_88 := 0;
   Spare_90 := 0;
   Spare_92 := 0;
   Spare_94 := 0;
   Spare_96 := 0;
   Spare_98 := 0;
   Spare_100 := 0;
   Spare_102 := 0;
   Spare_104 := 0;
   Spare_106 := 0;
   Spare_108 := 0;
   Spare_110 := 0;
   Spare_112 := 0;
   Spare_114 := 0;
   Spare_116 := 0;
   Spare_118 := 0;
   Spare_120 := 0;
   Spare_122 := 0;
   Spare_124 := 0;
   Spare_126 := 0;
   Spare_128 := 0;
   Spare_130 := 0;
   Spare_132 := 0;
   Spare_134 := 0;
   Spare_136 := 0;
   Spare_138 := 0;
   Spare_140 := 0;
   Spare_142 := 0;
   Spare_144 := 0;
   Spare_146 := 0;
   Spare_148 := 0;
   Spare_150 := 0;
   Spare_152 := 0;
   Spare_154 := 0;
   Spare_156 := 0;
   Spare_158 := 0;
   Spare_160 := 0;
   Spare_162 := 0;
   Spare_164 := 0;
   Spare_166 := 0;
   Spare_168 := 0;
   Spare_170 := 0;
   Spare_172 := 0;
   Spare_174 := 0;
   Spare_176 := 0;
   Spare_178 := 0;
   Spare_180 := 0;
   Spare_182 := 0;
   Spare_184 := 0;
   Spare_186 := 0;
   Spare_188 := 0;
   Spare_190 := 0;
   Spare_192 := 0;
   Spare_194 := 0;
   Spare_196 := 0;
   Spare_198 := 0;
   Spare_200 := 0;
   Spare_202 := 0;
   Spare_204 := 0;
   Spare_206 := 0;
   Spare_208 := 0;
   Spare_210 := 0;
   Spare_212 := 0;
   Spare_214 := 0;
   Spare_216 := 0;
   Spare_218 := 0;
   Spare_220 := 0;
   Spare_222 := 0;
   Spare_224 := 0;
   Spare_226 := 0;
   Spare_228 := 0;
   Spare_230 := 0;
   Spare_232 := 0;
   Spare_234 := 0;
   Spare_236 := 0;
   Spare_238 := 0;
   Spare_240 := 0;
   Spare_242 := 0;
   Spare_244 := 0;
   Spare_246 := 0;
   Spare_248 := 0;
   Spare_250 := 0;
   Spare_252 := 0;
   Spare_254 := 0;
   Spare_256 := 0;
   Spare_258 := 0;
   Spare_260 := 0;
   Spare_262 := 0;
   Spare_264 := 0;
   Spare_266 := 0;
   Spare_268 := 0;
   Spare_270 := 0;
   Spare_272 := 0;
   Spare_274 := 0;
   Spare_276 := 0;
   Spare_278 := 0;
   Spare_280 := 0;
   Spare_282 := 0;
   Spare_284 := 0;
   Spare_286 := 0;
   Spare_288 := 0;
   Spare_290 := 0;
   Spare_292 := 0;
   Spare_294 := 0;
   Spare_296 := 0;
   Spare_298 := 0;
END_DATA_BLOCK

